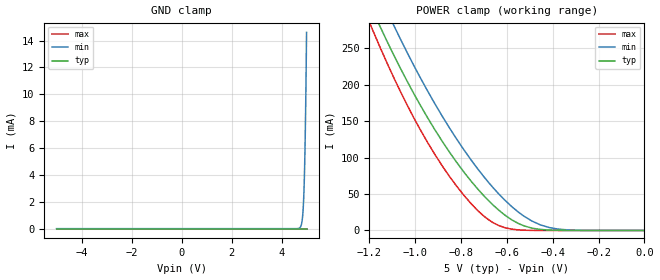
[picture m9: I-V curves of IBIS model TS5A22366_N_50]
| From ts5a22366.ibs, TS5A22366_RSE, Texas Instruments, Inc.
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[Model]   TS5A22366_N_50
Model_type  Terminator
| variable   typ   min   max
C_comp   38.27pF   34.21pF   41.92pF
| C_tri-state   38.27pF   34.21pF   41.92pF
[Temperature Range]   40   100   -40
| Ambient temperature   25   85   -40
[Voltage range]   5   4.5   5.5
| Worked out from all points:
|   POWER clamp passes 1 mA (typ) near -0.43 V on its own axis
[GND Clamp]
| TS5A22366_N_50
|   Voltage   I(typ)   I(min)   I(max)
-5V       -1.685nA   -158.2nA   -316.4pA
4.725V    677.6pA    58.23uA    48.53pA
4.785V    688.6pA    252.8uA    50.31pA
4.83V     697.5pA    706.2uA    51.64pA
4.865V    706.5pA    1.5mA      52.68pA
4.895V    719.8pA    2.745mA    53.57pA
4.91V     731.6pA    3.646mA    54.01pA
4.925V    750.5pA    4.777mA    54.46pA
4.95V     815.2pA    7.242mA    55.2pA
4.975V    978.9pA    10.51mA    55.94pA
4.985V    1.102nA    12.05mA    56.23pA
5V        1.403nA    14.6mA     56.68pA
[POWER Clamp]
| TS5A22366_N_50
|   Voltage   I(typ)   I(min)   I(max)
-5V       5.806A     5.781A     6.479A
-1.185V   301.5mA    344.2mA    274.6mA
-1.155V   280.9mA    323mA      252.5mA
-1.095V   241.6mA    282.4mA    210.7mA
-1.065V   222.8mA    262.9mA    191mA
-980mV    173.1mA    210.9mA    139.5mA
-880mV    121.4mA    155.7mA    87.65mA
-755mV    67.27mA    96.26mA    36.46mA
-660mV    34.85mA    58.66mA    10.71mA
-550mV    9.612mA    25.25mA    807.9uA
-415mV    552.6uA    3.996mA    7.74uA
0V        0A         0A         0A
